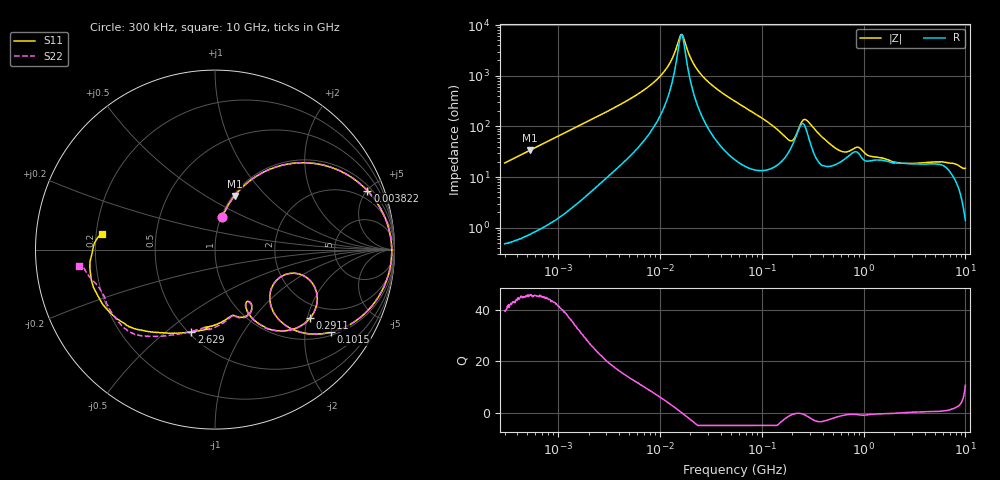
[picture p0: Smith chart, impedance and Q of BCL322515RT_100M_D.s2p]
! S-Parameter Data Generated by TDK Corporation
! Copyright(C) 2024 TDK Corporation.
! All Rights Reserved.
! TDK P/N: BCL322515RT-100M-D (SMD / SMT Inductor (Coil))
! Property: L=10uH at 1MHz
! Size(LxWxT): 3.2x2.5x1.5mm
! Model Type: s2p (Touchstone File Format Version 1.0)
! Frequency: DC=Yes Start=0.3MHz Stop=10000MHz 802points Log-sweep
! Model Generated on May 28, 2024
! Terms and conditions regarding TDK Simulation Models:
! 1)This simulation model is being provided solely for informational
!  purposes. Please refer to the specifications of the products in
!  terms of detailed characteristics of such products.
! 2)In no event shall TDK Corporation of any of its subsidiaries be
!  liable for any loss or damage arising, directly or indirectly,
!  from any information contained in this simulation model, including,
!  but not limited to loss or damages arising from any inaccuracies,
!  omissions or errors in connection with such information.
! 3)Any and all copyrights on this simulation model are owned by
!  TDK Corporation.  Duplication or redistribution of this simulation
!  model without prior written permission from TDK Corporation
!  is prohibited.
! 4)This simulation model is subject to any modification or change
!  without any prior notice.
! 5)Neither TDK Corporation nor any of its subsidiaries shall make any
!  warranty, express or implied, including but not limited to the
!  correctness, implied warranties of merchantability and fitness for
!  a particular purpose with respect to this simulation models.
! 6)The use of this simulation model shall be deemed to have consented
!  to the terms and conditions hereof.
! Port Assignments:
!  1 ---@@@--- 2
! Applicable Conditions:
!  Temperature = 25 degC
!  DC Bias Current = 0 A
!  Small Signal Operation
# Hz S MA R 50
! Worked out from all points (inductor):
!   801 points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, 300 kHz to 10 GHz, reference 50 ohm
!   read as one part in series: L = 10.1 uH near 318.3 kHz
!   highest Q = 45.6 at 536 kHz (marker M1), where L = 10.1 uH
!   self-resonance near 16.27 MHz
!   S11 on the Smith chart (normalised r, x): 300 kHz: 1.01, +0.38; 3.822 MHz: 1.31, +5.03; 101.5 MHz: 1.10, -2.74; 291.1 MHz: 1.58, -2.09; 2.629 GHz: 0.52, -0.62; 10 GHz: 0.22, +0.07
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300000  0.1834 77.7  0.9781 -10.8  0.9783 -10.7  0.1836 77.7
535999  0.3179 70.0  0.9408 -18.7  0.9412 -18.7  0.3179 70.0
1713600  0.7248 41.6  0.6652 -46.5  0.6656 -46.5  0.725 41.6
3822232  0.9104 21.1  0.3631 -65.5  0.3634 -65.4  0.9103 21.1
9671944  0.9774 5.9  0.1092 -75.3  0.1092 -75.3  0.9775 5.9
1.257005e7  0.9828 2.7  0.0551 -70.8  0.05512 -70.8  0.983 2.7
1.649435e7  0.9849 -0.6  0.01511 5.6  0.01512 5.6  0.985 -0.6
2.504582e7  0.9811 -5.7  0.08903 74.5  0.08908 74.5  0.9812 -5.8
5.477226e7  0.9342 -18.8  0.2977 67.2  0.2978 67.2  0.9342 -18.9
1.014901e8  0.7936 -35.4  0.5404 49.3  0.5406 49.3  0.7934 -35.5
1.405283e8  0.6245 -45.6  0.6754 33.8  0.6755 33.9  0.6243 -45.7
1.833272e8  0.417 -42.8  0.7163 15.6  0.7165 15.6  0.4165 -42.8
2.289088e8  0.4734 -16.3  0.5395 2.0  0.5398 2.0  0.4731 -16.3
2.910637e8  0.6529 -35.6  0.5147 27.2  0.5149 27.2  0.6538 -35.5
3.126428e8  0.6367 -42.4  0.5849 28.0  0.5851 28.0  0.6379 -42.3
5.285151e8  0.3896 -62.3  0.7881 6.8  0.7884 6.8  0.394 -62.4
8.528959e8  0.3902 -58.4  0.7125 -4.9  0.7128 -4.9  0.3934 -58.8
1.767019e9  0.4221 -90.7  0.7384 -23.5  0.7386 -23.5  0.4282 -88.6
2.629198e9  0.4779 -105.9  0.7061 -38.0  0.7065 -38.1  0.475 -106.2
6.333834e9  0.6654 -144.2  0.4997 -78.5  0.4999 -78.7  0.6728 -143.3
8.322921e9  0.7068 -168.8  0.4292 -100.9  0.4298 -101.0  0.6945 -164.6
1e10  0.6379 172.2  0.3392 -112.3  0.3388 -112.4  0.7624 -173.0
